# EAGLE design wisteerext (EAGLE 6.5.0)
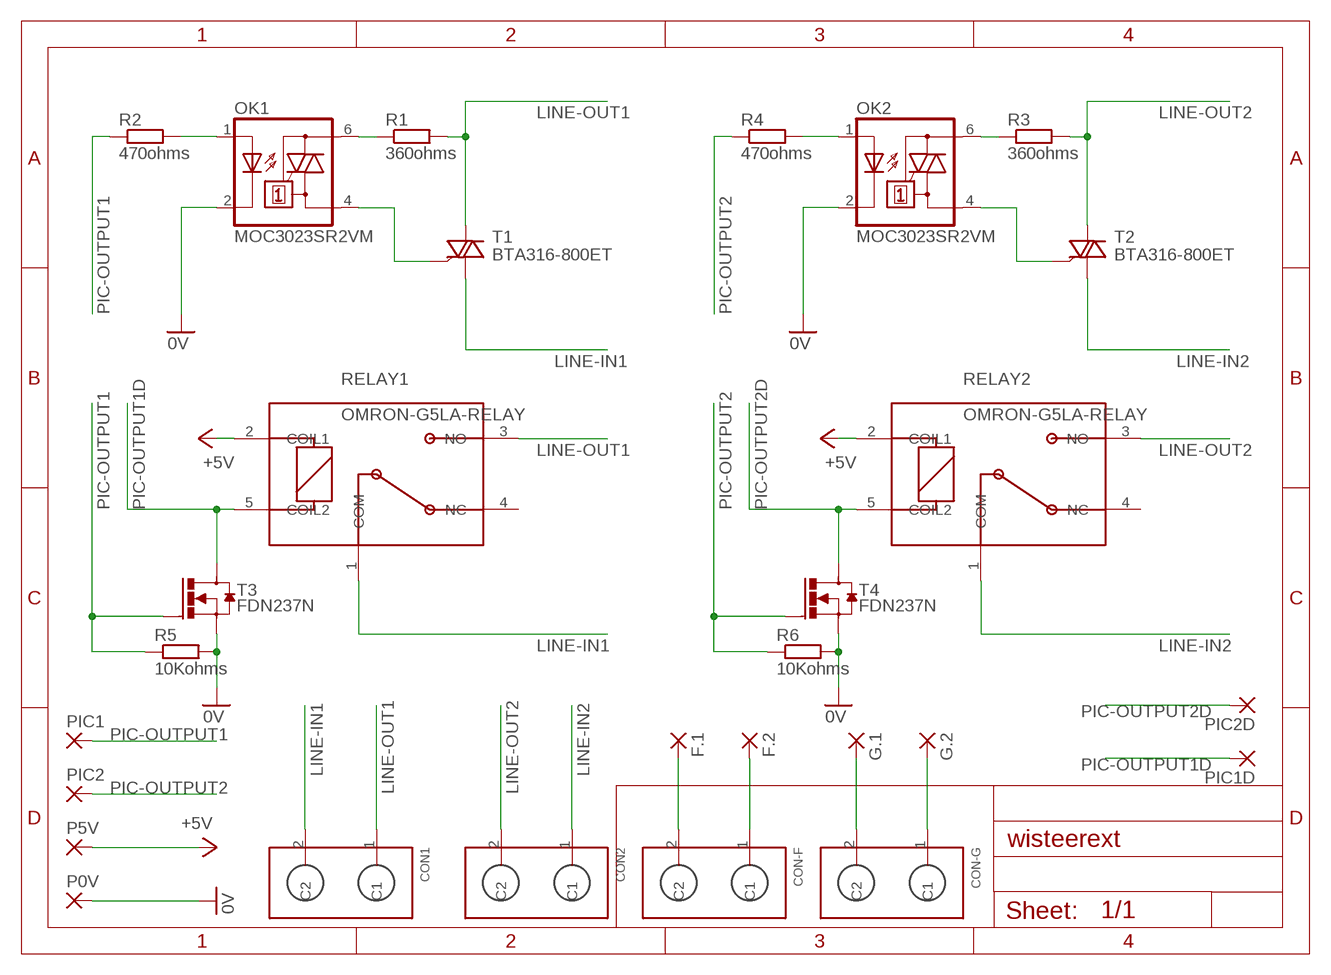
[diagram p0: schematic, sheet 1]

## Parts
CON1  SCREW-TERMINATION-X2  [PM5.08-2-90]
CON2  SCREW-TERMINATION-X2  [PM5.08-2-90]
CON-F  SCREW-TERMINATION-X22.54  [MPT0.5-2-2.54]
CON-G  SCREW-TERMINATION-X22.54  [MPT0.5-2-2.54]
F.1  1,6/0,8  [1,6/0,8]
F.2  1,6/0,8  [1,6/0,8]
G.1  1,6/0,8  [1,6/0,8]
G.2  1,6/0,8  [1,6/0,8]
OK1  MOC3023SR2VM  MOC3031S  [DIL6-SMD]
OK2  MOC3023SR2VM  MOC3031S  [DIL6-SMD]
P0V  2,54/0,9  [2,54/0,9]
P5V  2,54/0,9  [2,54/0,9]
PIC1  2,54/0,9  [2,54/0,9]
PIC1D  2,54/0,9  [2,54/0,9]
PIC2  2,54/0,9  [2,54/0,9]
PIC2D  2,54/0,9  [2,54/0,9]
R1  360ohms  R-EU_R2512  [R2512]
R2  470ohms  R-EU_R0603  [R0603]
R3  360ohms  R-EU_R2512  [R2512]
R4  470ohms  R-EU_R0603  [R0603]
R5  10Kohms  R-EU_R0603  [R0603]
R6  10Kohms  R-EU_R0603  [R0603]
RELAY1  OMRON-G5LA-RELAY  [OMRON-G5LA-RELAY]
RELAY2  OMRON-G5LA-RELAY  [OMRON-G5LA-RELAY]
T1  BTA316-800ET  [SOT78A]
T2  BTA316-800ET  [SOT78A]
T3  FDN237N  [SUPERSOT-3]
T4  FDN237N  [SUPERSOT-3]

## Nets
0V: OK1.2(C) OK2.2(C) P0V.1(P) R5.2 R6.2 T3.2(S) T4.2(S)
+5V: P5V.1(P) RELAY1.2(COIL1) RELAY2.2(COIL1)
LINE-IN1: CON1.2(C2) RELAY1.1(COM) T1.T1(CM)
LINE-IN2: CON2.1(C1) RELAY2.1(COM) T2.T1(CM)
LINE-OUT1: CON1.1(C1) R1.2 RELAY1.3(NO) T1.T2(LD)
LINE-OUT2: CON2.2(C2) R3.2 RELAY2.3(NO) T2.T2(LD)
N$1: OK1.4(A1) T1.G
N$2: OK1.6(A2) R1.1
N$3: OK2.4(A1) T2.G
N$4: OK1.1(A) R2.2
N$5: OK2.6(A2) R3.1
N$6: OK2.1(A) R4.2
N$7: CON-F.2(C2) F.1.1(P)
N$8: CON-F.1(C1) F.2.1(P)
N$9: CON-G.2(C2) G.1.1(P)
N$10: CON-G.1(C1) G.2.1(P)
PIC-OUTPUT1: PIC1.1(P) R2.1 R5.1 T3.1(G)
PIC-OUTPUT1D: PIC1D.1(P) RELAY1.5(COIL2) T3.3(D)
PIC-OUTPUT2: PIC2.1(P) R4.1 R6.1 T4.1(G)
PIC-OUTPUT2D: PIC2D.1(P) RELAY2.5(COIL2) T4.3(D)
Unconnected: RELAY1.4(NC) RELAY2.4(NC)

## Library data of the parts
CON1 CON2 CON-F CON-G = comps for wipee:SCREW-TERMINATION-X2: PM5.08-2-90 5.08mm spacement
F.1 F.2 G.1 G.2 = wirepad:1,6/0,8: THROUGH-HOLE PAD
OK1 OK2 = optocoupler:MOC30*: 6-Pin DIP Zero-Cross Optoisolators Triac Driver Output (250/400 Volt Peak) Source: The old path of data sheet not more available 2013-05-06.; MF: FAIRCHILD SEMICONDUCTOR; MPN: MOC3031SM; OC_FARNELL: unknown; OC_NEWARK: 34C1335
P0V P5V PIC1 PIC1D PIC2 PIC2D = wirepad:2,54/0,9: THROUGH-HOLE PAD
R1-R6 = rcl:R-EU_: RESISTOR, European symbol
RELAY1 RELAY2 = comps for wipee:OMRON-G5LA-RELAY: OMRON-G5LA-RELAY 5v, SPDT, 0.36W http://radiospares-fr.rs-online.com/web/p/relais-sans-accrochage/6839138/
T1 T2 = nxp_60_1_1:BTA316: Planar passivated high commutation three quadrant triac in a SOT78 plastic package intended for use in circuits where high static and dynamic dV/dt and high dI/dt can occur AAL Eindhoven MV+ MK; 12NC: 9340 646 19127
T3 T4 = mmm:FDN237N: MOSFET CANAL N FDN237N Fairchild semiconductors http://docs-europe.electrocomponents.com/webdocs/0d23/0900766b80d23106.pdf

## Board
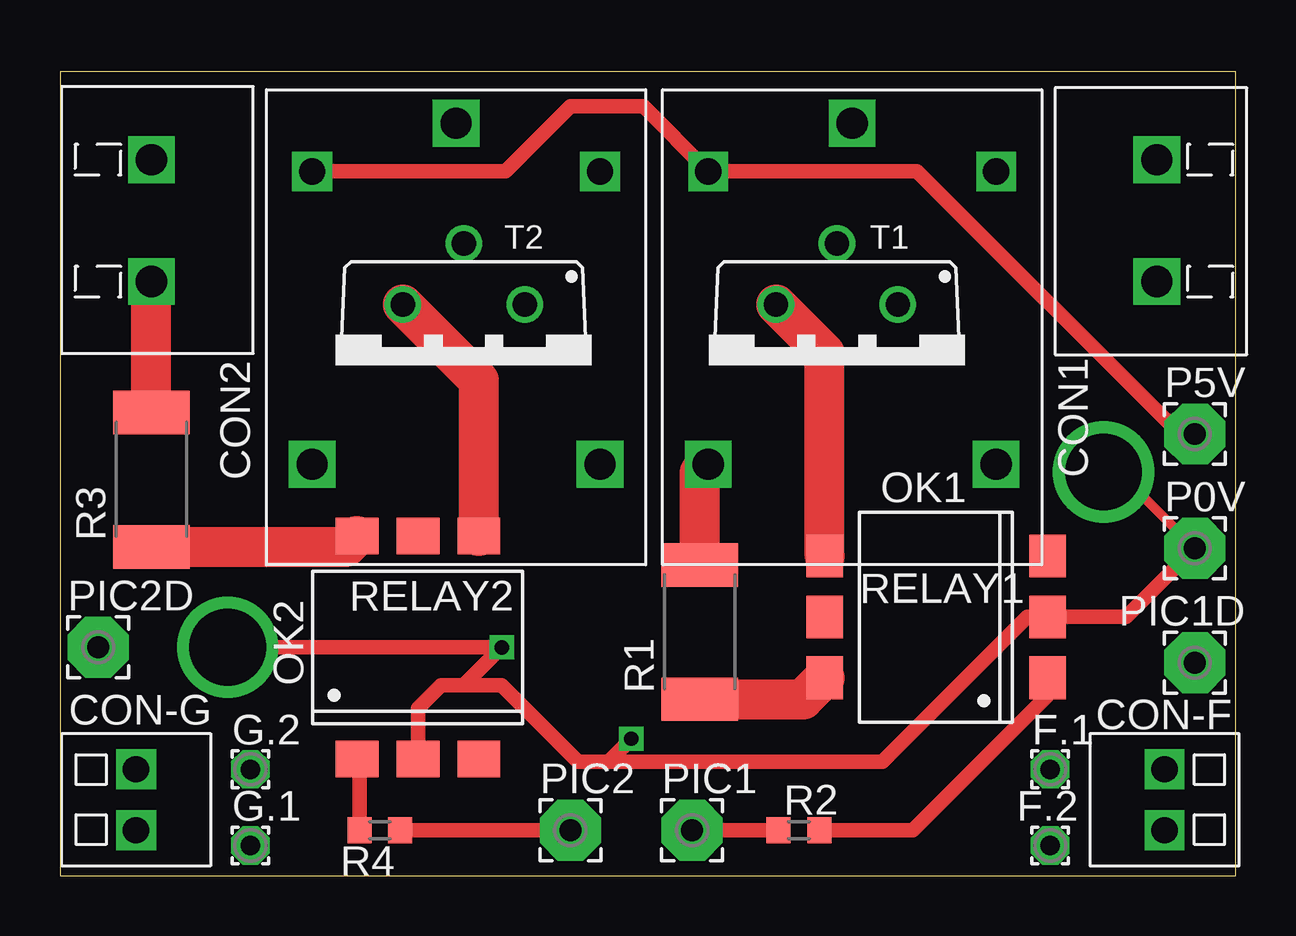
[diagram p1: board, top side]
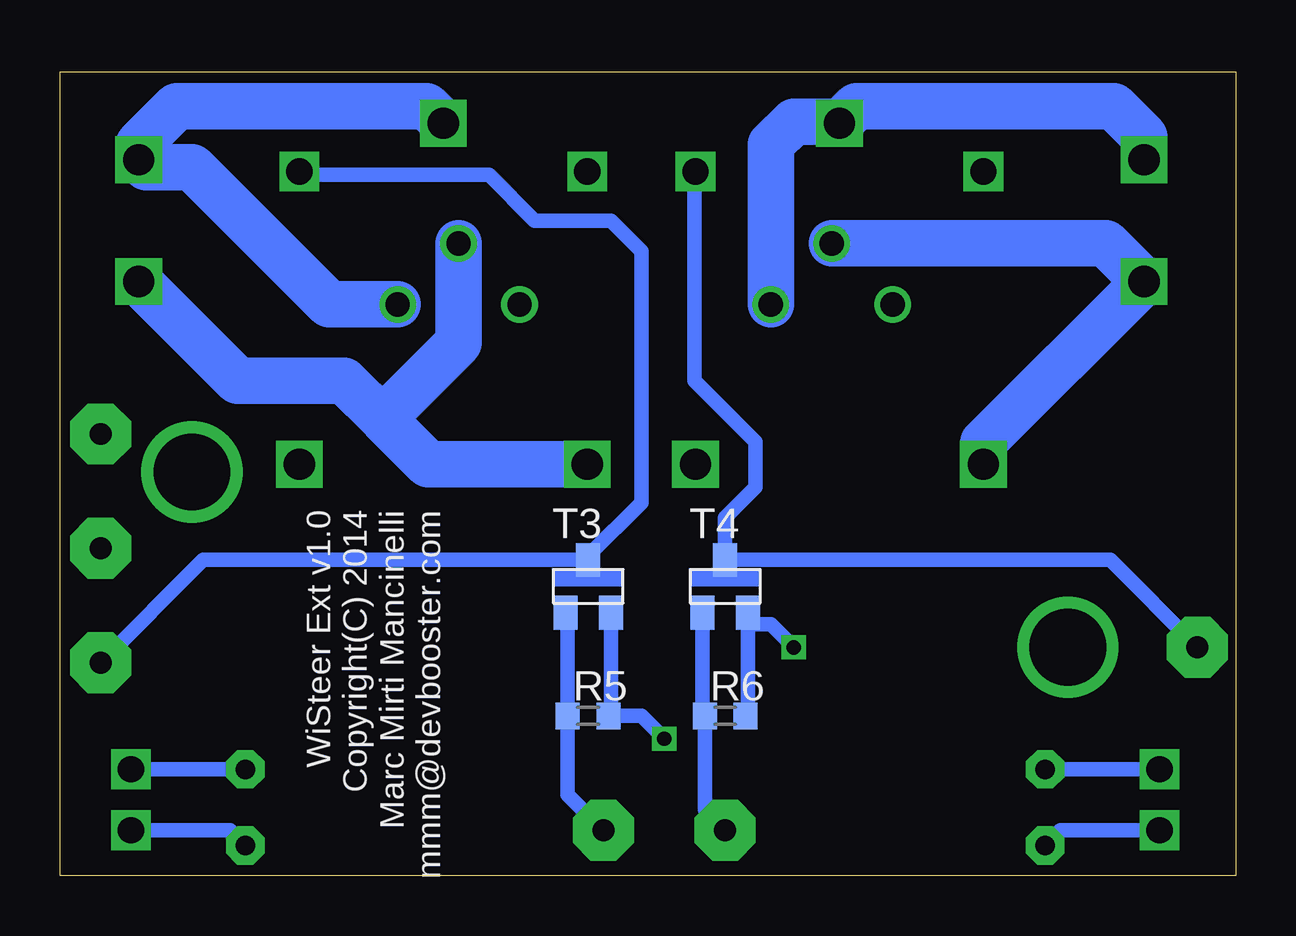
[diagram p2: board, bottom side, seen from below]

Size 49 x 33.5 mm. Coordinates in mm from the lower left corner, seen from the top.
Outline: 0,0 49,0 49,33.5 0,33.5 0,0
Copper layers (1*16): Top 0.035mm / dielectric 1.5mm / Bottom 0.035mm
Design rules "default *": minimum track width 10mil, minimum drill 12mil, track to track 8mil, track to pad 8mil, pad to pad 8mil, via to via 8mil, smd to smd 8mil, copper to edge 12mil, drill to drill 8mil, minimum pad ring 10mil, minimum via ring 8mil, stop-mask expansion 4mil, vias tented up to drill 0mil, thermal gap 10mil

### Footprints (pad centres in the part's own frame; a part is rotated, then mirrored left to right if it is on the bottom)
PM5.08-2-90 = drill 1.3 square: 1 -2.54,0; 2 2.54,0
MPT0.5-2-2.54 = drill 1.1 square: 1 -1.27,0; 2 1.27,0
1,6/0,8 = drill 0.813 pad 1.6 octagon: 1 0,0
DIL6-SMD = smd 1.78 x 1.52: 1 -2.54,-4.645; 2 0,-4.645; 3 2.54,-4.645; 4 2.54,4.645; 5 0,4.645; 6 -2.54,4.645
2,54/0,9 = drill 0.914 pad 2.54 octagon: 1 0,0
R2512 = smd 1.8 x 3.2: 1 -2.8,0; 2 2.8,0
R0603 = smd 1 x 1.1: 1 -0.85,0; 2 0.85,0
OMRON-G5LA-RELAY = drill 1.3 square: 1 -8.5,0; 3 5.7,-6; 4 5.7,6 | drill 1.1 square: 2 -6.5,-6; 5 -6.5,6
SOT78A = drill 1.016: G 2.54,0; T1 -2.54,0; T2 0,-2.54
SUPERSOT-3 = smd 1 x 1.4: 1 -0.95,-1.1; 2 0.95,-1.1; 3 0,1.1

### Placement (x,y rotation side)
CON1  45.72,27.3 90 top
CON2  3.81,27.3 270 top
CON-F  46.04,3.17 90 top
CON-G  3.17,3.17 270 top
F.1  41.27,4.45 0 top
F.2  41.27,1.27 0 top
G.1  7.94,1.27 0 top
G.2  7.94,4.45 0 top
OK1  36.51,10.79 90 top
OK2  14.92,9.53 0 top
P0V  47.31,13.65 0 top
P5V  47.31,18.41 0 top
PIC1  26.35,1.91 0 top
PIC1D  47.31,8.89 0 top
PIC2  21.27,1.91 0 top
PIC2D  1.59,9.53 0 top
R1  26.67,10.16 90 top
R2  30.8,1.91 0 top
R3  3.81,16.51 90 top
R4  13.34,1.91 180 top
R5  26.99,6.67 0 bottom
R6  21.27,6.67 0 bottom
RELAY1  33.02,22.86 270 top
RELAY2  16.51,22.86 270 top
T1  32.38,23.81 180 top
T2  16.83,23.81 180 top
T3  26.99,12.06 0 bottom
T4  21.27,12.06 0 bottom

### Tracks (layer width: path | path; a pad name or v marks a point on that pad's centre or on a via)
0V  (via drill 0.6, 3.2)
  Top 0.406: v43.5,16.83 44.13,16.83 P0V.1
  Top 0.61: 22.86,4.76 34.29,4.76 40.32,10.79 OK1.2 44.45,10.79 P0V.1 | 22.86,4.76 21.59,4.76 18.41,7.94 16.83,7.94 | 16.83,7.94 15.88,7.94 14.92,6.99 OK2.2 | 16.83,7.94 v18.41,9.53 v6.99,9.53 | v23.81,5.71 22.86,4.76
  Bottom 0.61: 26.04,6.77 R5.2 | T4.2 20.32,10.47 | R6.2 20.32,6.77 20.32,10.47 | 26.04,6.77 T3.2 | 26.04,6.77 26.04,6.67 24.77,6.67 v23.81,5.71 | 20.32,10.47 20.32,10.48 19.37,10.48 v18.41,9.53
+5V
  Top 0.61: RELAY2.2 18.57,29.36 21.27,32.07 24.31,32.07 RELAY1.2 35.73,29.36 46.67,18.41 P5V.1
LINE-IN1
  Bottom 1.93: RELAY1.1 33.73,32.07 44.13,32.07 45.72,30.48 CON1.2 45.4,29.53 43.5,29.53 37.78,23.81 T1.T1
LINE-IN2
  Bottom 1.93: CON2.1 3.81,30.8 5.08,32.07 15.8,32.07 RELAY2.1 16.58,31.43 18.41,31.43 19.37,30.48 T2.T1
LINE-OUT1
  Top 1.676: R1.2 26.67,16.81 RELAY1.3
  Bottom 1.93: 35.56,19.05 33.66,17.14 27.04,17.14 RELAY1.3 | T1.T2 32.38,22.23 35.56,19.05 | 35.56,19.05 37.15,20.64 41.59,20.64 CON1.1
LINE-OUT2
  Top 1.676: R3.2 CON2.2
  Bottom 1.93: RELAY2.3 10.51,18.07 CON2.2 5.4,26.35 T2.T2
N$1
  Top 1.676: OK1.4 31.87,21.79 T1.G
N$2
  Top 1.676: R1.1 30.97,7.36 OK1.6
N$3
  Top 1.676: OK2.4 17.46,20.64 T2.G
N$4
  Top 0.61: OK1.1 41.16,7.5 35.56,1.91 R2.2
N$5
  Top 1.676: R3.1 11.92,13.71 OK2.6
N$6
  Top 0.61: R4.2 12.48,4.78 OK2.1
N$7
  Bottom 0.61: CON-F.2 F.1.1
N$8
  Bottom 0.61: CON-F.1 41.91,1.91 F.2.1
N$9
  Bottom 0.61: CON-G.2 7.3,1.91 G.1.1
N$10
  Bottom 0.61: CON-G.1 G.2.1
PIC-OUTPUT1
  Top 0.61: R2.1 PIC1.1
  Bottom 0.61: T3.1 27.84,10.87 R5.1 27.84,3.39 PIC1.1
PIC-OUTPUT1D
  Bottom 0.61: RELAY1.5 38.87,29.21 31.11,29.21 29.21,27.3 26.04,27.3 24.77,26.04 24.77,15.56 26.99,13.34 T3.3 43.03,13.16 PIC1D.1
PIC-OUTPUT2
  Top 0.61: R4.1 PIC2.1
  Bottom 0.61: T4.1 22.22,6.77 R6.1 22.12,2.75 PIC2.1
PIC-OUTPUT2D
  Bottom 0.61: RELAY2.5 22.54,29.33 22.54,20.64 20,18.1 20,16.19 21.27,14.92 T4.3 5.23,13.16 PIC2D.1

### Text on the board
bNames: WiSteer Ext v1.0 / Copyright(C) 2014 / Marc Mirti Mancinelli / mmm@devbooster.com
